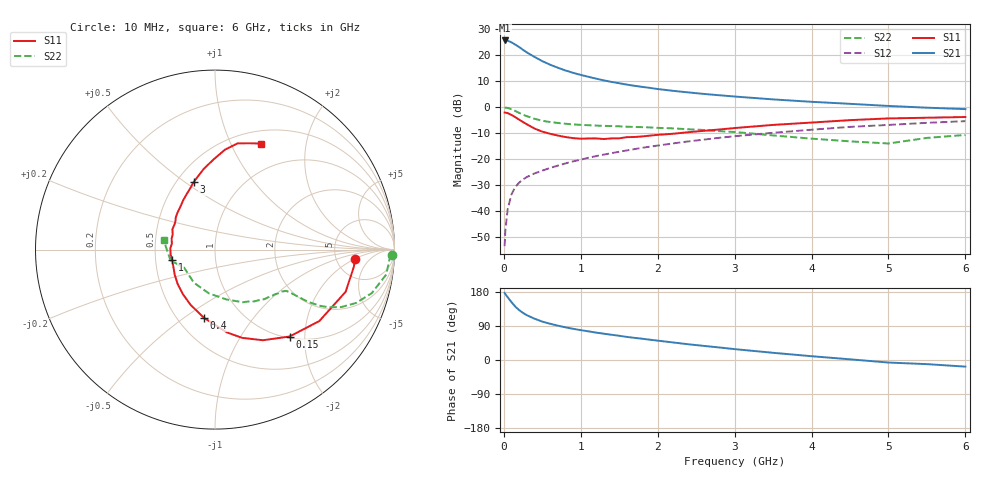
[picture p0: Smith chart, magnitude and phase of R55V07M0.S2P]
! SIEMENS Small Signal Semiconductors
! BFR183
! Si NPN RF Bipolar Junction Transistor in SOT23
! VCE = 5 V  IC = 7 mA
! Common Emitter S-Parameters:  May  1996
# GHz  S  MA  R  50
!  f  S11  S21  S12  S22
! GHz  MAG  ANG  MAG  ANG  MAG  ANG  MAG  ANG
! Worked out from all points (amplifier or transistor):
!   36 points, 10 MHz to 6 GHz, reference 50 ohm
!   highest |S21| = 25.6 dB at 10 MHz (marker M1)
!   |S21| within 3 dB of that: start of sweep to 221 MHz
!   unconditionally stable (mu >= 1): 910.2 MHz to 2.623 GHz
!   at 250 MHz: K = 0.51, MSG = 24.9 dB, |S12| = -27.8 dB
!   at 1.4 GHz: K = 1.06, MAG = 12.3 dB, |S12| = -17.7 dB
!   at 6 GHz: K = 0.88, MSG = 2.3 dB, |S12| = -5.4 dB
!   lowest NFmin = 1.25 dB at 450 MHz
!   S11 on the Smith chart (normalised r, x): 10 MHz: 7.67, -2.00; 150 MHz: 1.03, -1.68; 400 MHz: 0.67, -0.60; 1 GHz: 0.61, -0.08; 3 GHz: 0.61, +0.54; 6 GHz: 0.65, +1.31
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0.01  0.7825 -3.7  19.16 177.0  0.0021 87.4  0.9848 -1.7
0.02  0.7794 -7.1  18.95 173.9  0.0043 88.3  0.9734 -3.3
0.05  0.7649 -17.9  18.93 165.5  0.0108 80.7  0.964 -8.3
0.1  0.7046 -34.4  17.62 152.6  0.021 73.0  0.9066 -15.5
0.15  0.6379 -49.4  15.88 140.6  0.0291 67.9  0.8407 -20.7
0.2  0.5714 -62.1  14.29 131.5  0.0352 64.7  0.7724 -24.5
0.25  0.5141 -73.0  12.62 124.2  0.0406 61.3  0.7122 -26.8
0.3  0.466 -81.8  11.26 118.1  0.0451 60.9  0.6671 -28.1
0.4  0.3856 -99.1  9.221 108.9  0.0529 59.3  0.5944 -29.3
0.5  0.3366 -113.8  7.654 101.3  0.0598 59.9  0.5447 -29.5
0.6  0.3063 -125.6  6.557 95.7  0.0672 59.9  0.5157 -29.6
0.8  0.2652 -147.6  5.075 86.3  0.0822 61.1  0.478 -29.8
1  0.2459 -166.0  4.157 78.8  0.0971 62.1  0.455 -30.4
1.1  0.2486 -174.3  3.821 75.6  0.1058 62.3  0.4473 -31.3
1.3  0.2426 172.1  3.263 69.4  0.1217 62.1  0.4348 -32.8
1.6  0.2632 154.3  2.704 60.9  0.1464 61.2  0.4189 -36.3
2.2  0.3064 129.2  2.054 46.3  0.1996 57.8  0.389 -45.3
3  0.3946 107.6  1.597 28.7  0.2748 50.4  0.3313 -62.3
3.5  0.4535 98.0  1.405 19.0  0.3198 44.7  0.2846 -77.2
4.5  0.5603 84.2  1.155 1.8  0.4156 32.8  0.2188 -122.5
5.5  0.6234 71.9  0.973 -10.9  0.4972 20.8  0.2548 -166.2
6  0.6439 66.5  0.913 -17.5  0.5358 13.0  0.2905 169.8
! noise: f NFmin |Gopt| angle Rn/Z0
0.45  1.25  0.18  42  0.22
0.9  1.3  0.22  110  0.2
1.8  2  0.33  180  0.14
